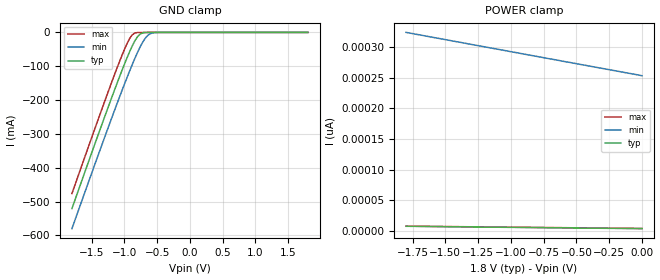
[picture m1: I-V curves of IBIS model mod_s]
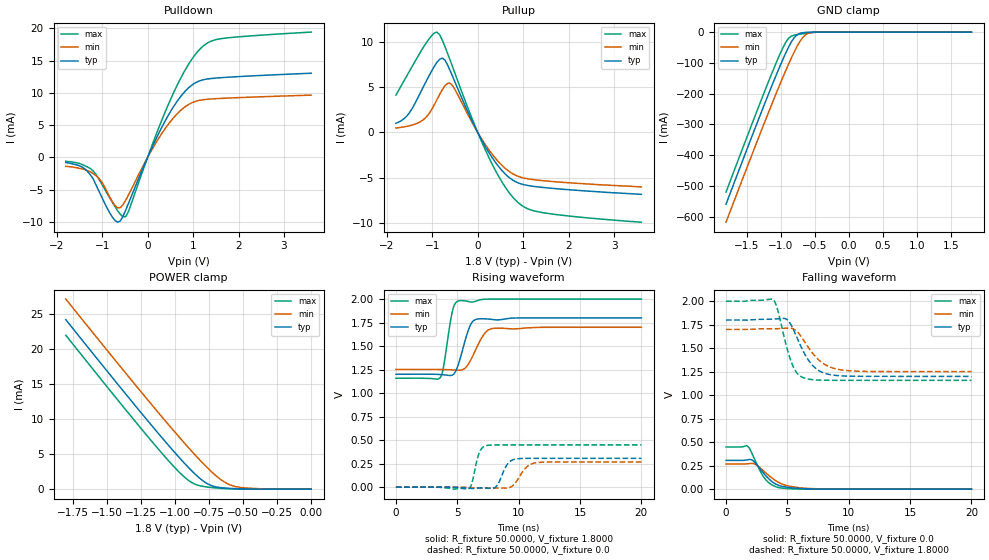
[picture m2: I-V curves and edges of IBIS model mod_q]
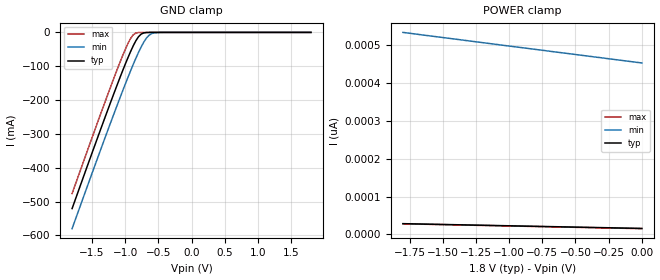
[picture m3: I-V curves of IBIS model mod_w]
| IBIS (I/O, Buffer, Information, Specification) Model, officially
| electronic behavioral standard for Buffer structures of digital pins.
[IBIS ver]  4.0
[File name] m95xxx_g7_tssop8.ibs
[File Rev]  1.0
[Date]   25 Aug 2015
[Source]   CAD & Design Services (Catania) - STMicroelectronics
[Notes]
   (Note1)  This IBIS model includes the TSSOP8 ceramic package parasitic data
   (Note2)  This IBIS model considers: VCC= 1.80(TYP), 1.70(MIN), 2.00(MAX)
   (Note3)  This IBIS model has some Notes about the non-monotonicity
   of the I-V curves, but they are not indicative of problems
   inside the model;
[Copyright] (c) 2015 STMicroelectronics
|   Component M95XXX
[Component] M95XXX
[Manufacturer] STMicroelectronics
[Package]
| variable   typ   min   max
R_pkg   0.0   0.0   0.0
L_pkg   0.0H   0.0H   0.0H
C_pkg   0.0F   0.0F   0.0F
[Pin]  signal_name   model_name   R_pin   L_pin   C_pin
1   SN   mod_s   NA   NA   NA
2   Q   mod_q   NA   NA   NA
3   WN   mod_w   NA   NA   NA
4   GND   GND   NA   NA   NA
5   D   mod_s   NA   NA   NA
6   C   mod_s   NA   NA   NA
7   HOLDN   mod_h   NA   NA   NA
8   VCCIO   POWER   NA   NA   NA
[Package Model]  182696_TSSOP8
[Define Package Model]  182696_TSSOP8
[Manufacturer]  STMicroelectronics
[OEM]  STMicroelectronics
[Description]  8 pin TSSOP package
[Number Of Pins]  8
[Pin Numbers]
|Pin Num   Terminal Name
1   | net1
2   | net2
3   | net3
4   | net4_GND
5   | net5
6   | net6
7   | net7
8   | net8_VDD
[Model Data]
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[End Model Data]
[End Package Model]
| Models and submodels in the file (4): mod_s (Input), mod_q (I/O), mod_w (Input), mod_h (Input)
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|   Model mod_s
[Model]   mod_s
Model_type Input
Vinl   =   0.540V
Vinh   =   1.260V
C_comp   2.119pF   2.023pF   2.323pF
[Temperature Range]   25.0000   0.1050k   -40.0000
[Voltage Range]   1.8000V   1.7000V   2.0000V
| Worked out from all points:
|   GND clamp passes 1 mA (typ) near -0.70 V on its own axis
[GND_clamp]
|Voltage   I(typ)   I(min)   I(max)
-1.8V     -520.9mA   -580.3mA   -476.5mA
-1.2V     -196.3mA   -256.7mA   -150.7mA
-1.04V    -114.2mA   -173.8mA   -69.64mA
-960mV    -75.5mA    -133.8mA   -33.44mA
-880mV    -40.19mA   -95.27mA   -7.262mA
-800mV    -12.93mA   -59.45mA   -437.7uA
-760mV    -5.115mA   -43.21mA   -157.1uA
-720mV    -1.573mA   -28.76mA   -100.4uA
-640mV    -132.4uA   -8.366mA   -67.87uA
-560mV    -24.53uA   -1.273mA   -44.38uA
-480mV    -7.538uA   -153uA     -22.96uA
1.8V      15.87pA    456.8pA    13.84pA
[POWER_clamp]
|Voltage   I(typ)   I(min)   I(max)
-1.8V     7.58pA     324.2pA    7.783pA
-700mV    5.176pA    280.9pA    5.483pA
-680mV    5.133pA    280.2pA    5.442pA
0V        3.691pA    253.5pA    4.042pA
|   Model mod_q
[Model]   mod_q
Model_type I/O
Polarity   Non-Inverting
Enable   Active-Low
Vinl   =   0.540V
Vinh   =   1.260V
Vmeas  =   0.900V
Cref   =   30pF
C_comp   3.207pF   3.063pF   3.358pF
[Temperature Range]   25.0000   0.1050k   -40.0000
[Voltage Range]   1.8000V   1.7000V   2.0000V
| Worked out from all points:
|   slope of the pulldown table from 0 to 0.27 V, typ, clamps not added: 66.3 ohm
|   slope of the pullup table from 0 to 0.27 V, typ, clamps not added: 112 ohm
|   GND clamp passes 1 mA (typ) near -0.63 V on its own axis
|   POWER clamp passes 1 mA (typ) near -0.78 V on its own axis
|   rising waveform, R_fixture 50.0000, V_fixture 1.8000: 20-80 % time 807ps typ, 1.05ns min, 597ps max; typ from 1.2 V to 1.8 V
|   rising waveform, R_fixture 50.0000, V_fixture 0.0: 20-80 % time 660ps typ, 873ps min, 489ps max; typ from 0 V to 0.306 V
|   falling waveform, R_fixture 50.0000, V_fixture 0.0: 20-80 % time 1.35ns typ, 1.7ns min, 1.13ns max; typ from 0.306 V to 0 V
|   falling waveform, R_fixture 50.0000, V_fixture 1.8000: 20-80 % time 1.48ns typ, 1.69ns min, 1.04ns max; typ from 1.8 V to 1.2 V
[Pulldown]
|Voltage   I(typ)   I(min)   I(max)
-1.8V     -800uA     -1.384mA   -600uA
-1.32V    -2.2mA     -2.06mA    -1.5mA
-1.02V    -5.99mA    -3.7mA     -3.98mA
-720mV    -9.764mA   -7.464mA   -7.616mA
-600mV    -9.857mA   -7.797mA   -8.83mA
-480mV    -8.145mA   -6.616mA   -9.19mA
60mV      953.5uA    767.3uA    1.16mA
420mV     6.082mA    4.799mA    7.619mA
780mV     9.899mA    7.607mA    12.98mA
1.14V     11.86mA    8.85mA     16.72mA
1.62V     12.37mA    9.153mA    18.42mA
3.6V      13.06mA    9.66mA     19.44mA
[Pullup]
|Voltage   I(typ)   I(min)   I(max)
-1.8V     1.015mA    496uA      4.135mA
-1.5V     2.197mA    745uA      6.809mA
-1.2V     5.018mA    1.401mA    9.404mA
-900mV    7.754mA    3.611mA    11.12mA
-780mV    8.236mA    4.734mA    10.23mA
-600mV    6.764mA    5.438mA    7.909mA
-180mV    1.872mA    1.633mA    2.241mA
180mV     -1.666mA   -1.441mA   -2.07mA
540mV     -4.257mA   -3.679mA   -5.541mA
840mV     -5.472mA   -4.756mA   -7.539mA
1.44V     -6.092mA   -5.345mA   -8.888mA
3.6V      -6.85mA    -6.03mA    -9.94mA
[GND_clamp]
|Voltage   I(typ)   I(min)   I(max)
-1.8V     -559.4mA   -618.2mA   -520.2mA
-1.2V     -214.3mA   -274.2mA   -173.7mA
-1.04V    -126.9mA   -186.2mA   -87.22mA
-960mV    -85.5mA    -143.6mA   -48.31mA
-880mV    -47.65mA   -102.7mA   -19.45mA
-800mV    -17.95mA   -64.52mA   -9.981mA
-760mV    -8.981mA   -47.2mA    -8.395mA
-720mV    -4.357mA   -31.76mA   -7.048mA
-640mV    -1.164mA   -9.757mA   -4.512mA
-560mV    -259.3uA   -1.789mA   -2.186mA
-440mV    -32.94uA   -178.6uA   -105.7uA
1.8V      87.14pA    73.75nA    65.36pA
[POWER_clamp]
|Voltage   I(typ)   I(min)   I(max)
-1.8V     24.23mA    27.18mA    22mA
-1.42V    15.03mA    18.01mA    12.77mA
-1.14V    8.405mA    11.38mA    6.161mA
-980mV    4.785mA    7.708mA    2.666mA
-880mV    2.694mA    5.497mA    984.9uA
-800mV    1.28mA     3.817mA    418.9uA
-740mV    571.4uA    2.65mA     251.7uA
-660mV    208.6uA    1.329mA    116.3uA
-580mV    94.3uA     506.2uA    41.18uA
-500mV    36.93uA    208.4uA    10.12uA
-360mV    1.708uA    50.12uA    81.12nA
0V        87.14pA    1.49nA     87.73pA
[Ramp]
| variable   typ   min   max
dV/dt_r   0.1836/0.7370n   0.1602/0.9802n   0.2693/0.5509n
dV/dt_f   0.3598/1.5225n   0.2693/1.7239n   0.5057/1.1750n
R_load = 50.0000
[Rising Waveform]
R_fixture= 50.0000
V_fixture= 1.8000
V_fixture_min= 1.7000
V_fixture_max= 2.0000
|time   V(typ)   V(min)   V(max)
0s        1.2V       1.251V     1.158V
3.63ns    1.197V     1.251V     1.167V
3.87ns    1.194V     1.25V      1.272V
4.62ns    1.193V     1.246V     1.88V
5.1ns     1.309V     1.243V     1.98V
5.94ns    1.682V     1.316V     1.972V
6.54ns    1.784V     1.473V     1.978V
7.26ns    1.79V      1.64V      1.999V
7.8ns     1.784V     1.686V     2V
20ns      1.8V       1.7V       2V
[Rising Waveform]
R_fixture= 50.0000
V_fixture= 0.0
V_fixture_min= 0.0
V_fixture_max= 0.0
|time   V(typ)   V(min)   V(max)
0s        3.52nV     163.6nV    3.442nV
5.91ns    -11.9mV    -4.13mV    -21.2mV
6.18ns    -15.05mV   -5.787mV   37.68mV
6.81ns    -9.41mV    -8.742mV   371.1mV
7.41ns    -10.99mV   -11.74mV   442.4mV
8.13ns    184.9uV    -10.36mV   448.3mV
9.09ns    244.5mV    -9.788mV   448.7mV
9.72ns    297.3mV    41.86mV    448.7mV
11.34ns   305.9mV    257.1mV    448.7mV
20ns      306mV      267.1mV    448.7mV
[Falling Waveform]
R_fixture= 50.0000
V_fixture= 0.0
V_fixture_min= 0.0
V_fixture_max= 0.0
|time   V(typ)   V(min)   V(max)
0s        306mV      267.1mV    448.7mV
1.74ns    311.6mV    270.2mV    459mV
2.205ns   301.7mV    272.6mV    353.7mV
2.745ns   220.5mV    230.8mV    203.7mV
3.135ns   158.9mV    185.1mV    117.4mV
3.585ns   97.74mV    134.5mV    57.86mV
4.305ns   39.42mV    70.15mV    16.15mV
5.205ns   16.62mV    30.78mV    4.807mV
7.185ns   2.061mV    5.038mV    209.2uV
20ns      -6.943nV   162.2nV    -29.02nV
[Falling Waveform]
R_fixture= 50.0000
V_fixture= 1.8000
V_fixture_min= 1.7000
V_fixture_max= 2.0000
|time   V(typ)   V(min)   V(max)
0s        1.8V       1.7V       2V
3.855ns   1.809V     1.707V     2.015V
4.17ns    1.813V     1.708V     1.925V
4.86ns    1.814V     1.712V     1.553V
5.34ns    1.738V     1.712V     1.345V
5.79ns    1.61V      1.677V     1.235V
6.33ns    1.458V     1.583V     1.184V
7.41ns    1.275V     1.393V     1.162V
9.21ns    1.207V     1.273V     1.158V
20ns      1.2V       1.251V     1.158V
|   Model mod_w
[Model]   mod_w
Model_type Input
Vinl   =   0.540V
Vinh   =   1.260V
C_comp   2.119pF   2.023pF   2.323pF
[Temperature Range]  25.0000   0.1050k   -40.0000
[Voltage Range]   1.8000V   1.7000V   2.0000V
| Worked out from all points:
|   GND clamp passes 1 mA (typ) near -0.70 V on its own axis
[GND_clamp]
|Voltage   I(typ)   I(min)   I(max)
-1.8V     -520.9mA   -580.3mA   -476.5mA
-1.2V     -196.3mA   -256.7mA   -150.7mA
-1.04V    -114.2mA   -173.8mA   -69.64mA
-960mV    -75.5mA    -133.8mA   -33.44mA
-880mV    -40.19mA   -95.27mA   -7.262mA
-800mV    -12.93mA   -59.45mA   -437.7uA
-760mV    -5.115mA   -43.21mA   -157.1uA
-720mV    -1.573mA   -28.76mA   -100.4uA
-640mV    -132.4uA   -8.366mA   -67.87uA
-560mV    -24.53uA   -1.273mA   -44.38uA
-480mV    -7.538uA   -153uA     -22.96uA
1.8V      15.87pA    456.8pA    13.84pA
[POWER_clamp]
|Voltage   I(typ)   I(min)   I(max)
-1.8V     28.44pA    533pA      28.05pA
-1.68V    27.59pA    527.5pA    27.19pA
-960mV    22.55pA    495.2pA    22.07pA
0V        15.87pA    452.4pA    15.26pA
